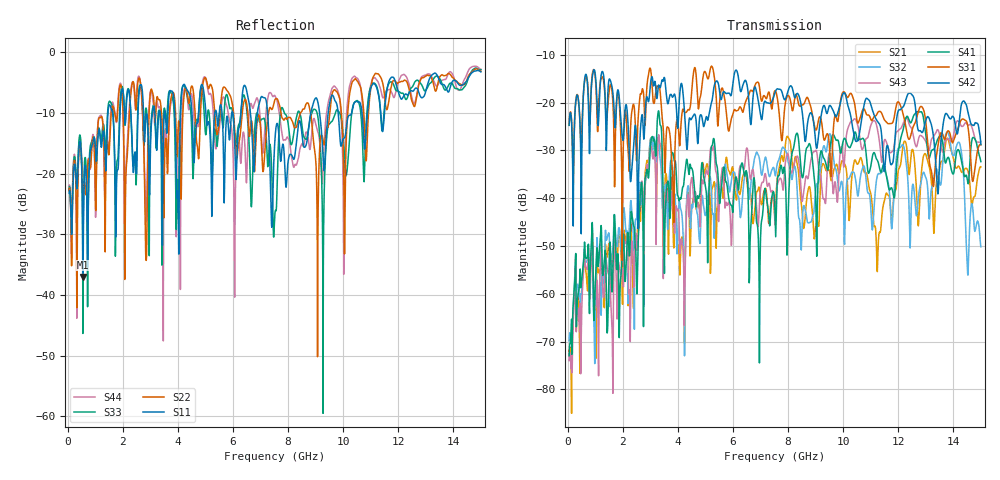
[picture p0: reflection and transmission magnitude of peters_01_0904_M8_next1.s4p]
# MHZ S RI R 50.00
! FREQ  S11  S12  S13  S14
!  S21  S22  S23  S24
!  S31  S32  S33  S34
!  S41  S42  S43  S44
!  REAL  IMAG  REAL  IMAG  REAL  IMAG  REAL  IMAG
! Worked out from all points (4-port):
!   1496 points, 50 MHz to 15 GHz, reference 50 ohm
!   strongest paths, dB at 50 MHz, 3.79 GHz, 7.53 GHz, 11.27 GHz, 15 GHz:
!     S42: -24.7, -18.8, -17.8, -24.1, -28.7
!     S31: -24.7, -33.0, -17.5, -21.9, -28.8
!     S41: -73.0, -30.4, -44.2, -32.5, -32.3
!     S43: -74.0, -38.4, -45.6, -26.3, -28.1
!     S32: -69.8, -33.3, -35.2, -34.9, -50.2
!     S21: -71.8, -39.9, -43.7, -50.1, -33.4
!   lowest |S11| = -37.0 dB at 550 MHz (marker M1), VSWR 1.03, Z = 49.1 - j1.02 ohm
!   |S11| at or under -10 dB: start of sweep to 1.46 GHz; 7.255 GHz to 8.824 GHz (1.568 GHz wide, 19.5 % of centre); 9.818 GHz to 10.31 GHz (494.9 MHz wide, 4.92 % of centre)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
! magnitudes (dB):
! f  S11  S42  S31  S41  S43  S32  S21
! 50 MHz  -23.2  -24.7  -24.7  -73.0  -74.0  -69.8  -71.8
! 550 MHz  -37.0  -20.7  -20.1  -54.9  -57.4  -54.6  -55.7
! 3.31 GHz  -10.0  -16.3  -16.6  -22.0  -26.8  -27.7  -27.4
! 4.21 GHz  -5.3  -19.6  -21.6  -37.2  -54.8  -52.0  -52.7
! 6.95 GHz  -8.6  -20.7  -16.3  -58.6  -42.5  -31.4  -37.7
! 8.31 GHz  -14.6  -18.2  -18.5  -26.4  -31.3  -36.3  -32.1
! 15 GHz  -3.3  -28.7  -28.8  -32.3  -28.1  -50.2  -33.4
